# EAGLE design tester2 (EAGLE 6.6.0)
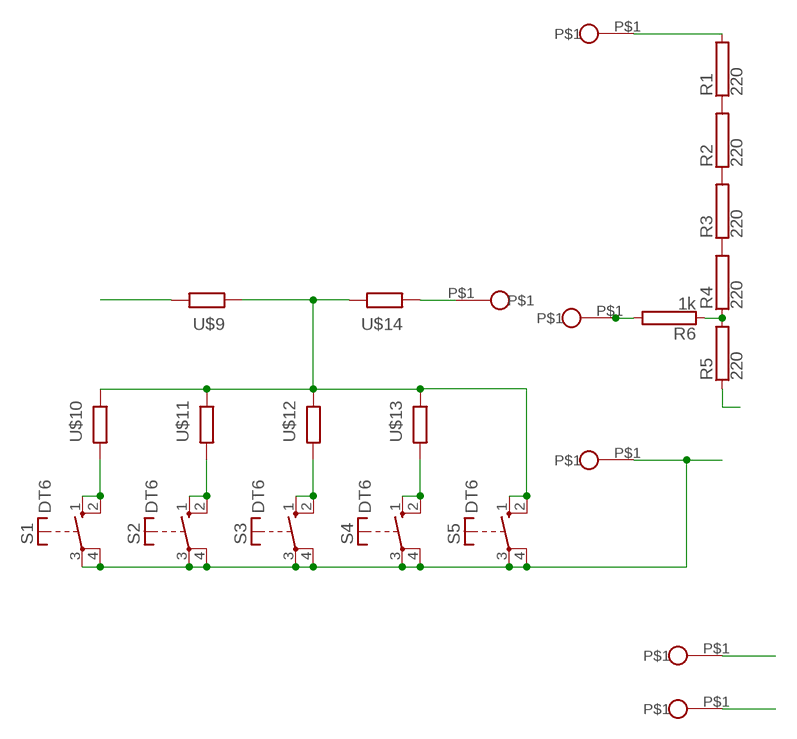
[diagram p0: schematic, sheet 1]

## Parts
R1  220  RCA5220  [CA5220]
R2  220  RCA5220  [CA5220]
R3  220  RCA5220  [CA5220]
R4  220  RCA5220  [CA5220]
R5  220  RCA5220  [CA5220]
R6  1k  RHPS923  [HPS923]
S1  DT6  [DT6]
S2  DT6  [DT6]
S3  DT6  [DT6]
S4  DT6  [DT6]
S5  DT6  [DT6]
U$2  PIN_N  [PIN_N]
U$3  PIN_N  [PIN_N]
U$6  PIN_N  [PIN_N]
U$8  PIN_N  [PIN_N]
U$9  R06W  [R06W2]
U$10  R06W  [R06W2]
U$11  R06W  [R06W2]
U$12  R06W  [R06W2]
U$13  R06W  [R06W2]
U$14  R06W  [R06W2]
U$16  PIN_N  [PIN_N]
U$17  PIN_N  [PIN_N]

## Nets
-UG: U$9.2
F1: U$16.P$1
F2: U$17.P$1
GND: S1.3(P) S1.4(P) S2.3(P) S2.4(P) S3.3(P) S3.4(P) S4.3(P) S4.4(P) S5.3(P) S5.4(P) U$6.P$1
N$1: R1.1 R2.2
N$2: R2.1 R3.2
N$3: R3.1 R4.2
N$4: R4.1 R5.2 R6.1
N$11: S1.1(S) S1.2(S) U$10.1
N$14: S2.1(S) S2.2(S) U$11.1
N$15: S3.1(S) S3.2(S) U$12.1
N$16: S4.1(S) S4.2(S) U$13.1
N$29: S5.1(S) S5.2(S) U$9.1 U$10.2 U$11.2 U$12.2 U$13.2 U$14.2
UA: R1.2 U$3.P$1
UB: R5.1
UG1: U$8.P$1 U$14.1
UG2: R6.2 U$2.P$1

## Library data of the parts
R1-R6 = resistor-power:R: Power Resitor; OC_FARNELL: unknown; OC_NEWARK: unknown
S1-S5 = switch-misc:DT: ITT SWITCH
U$2 U$3 U$6 U$8 U$16 U$17 = lampy02:PIN_N
U$9-U$14 = lampy02:R06W

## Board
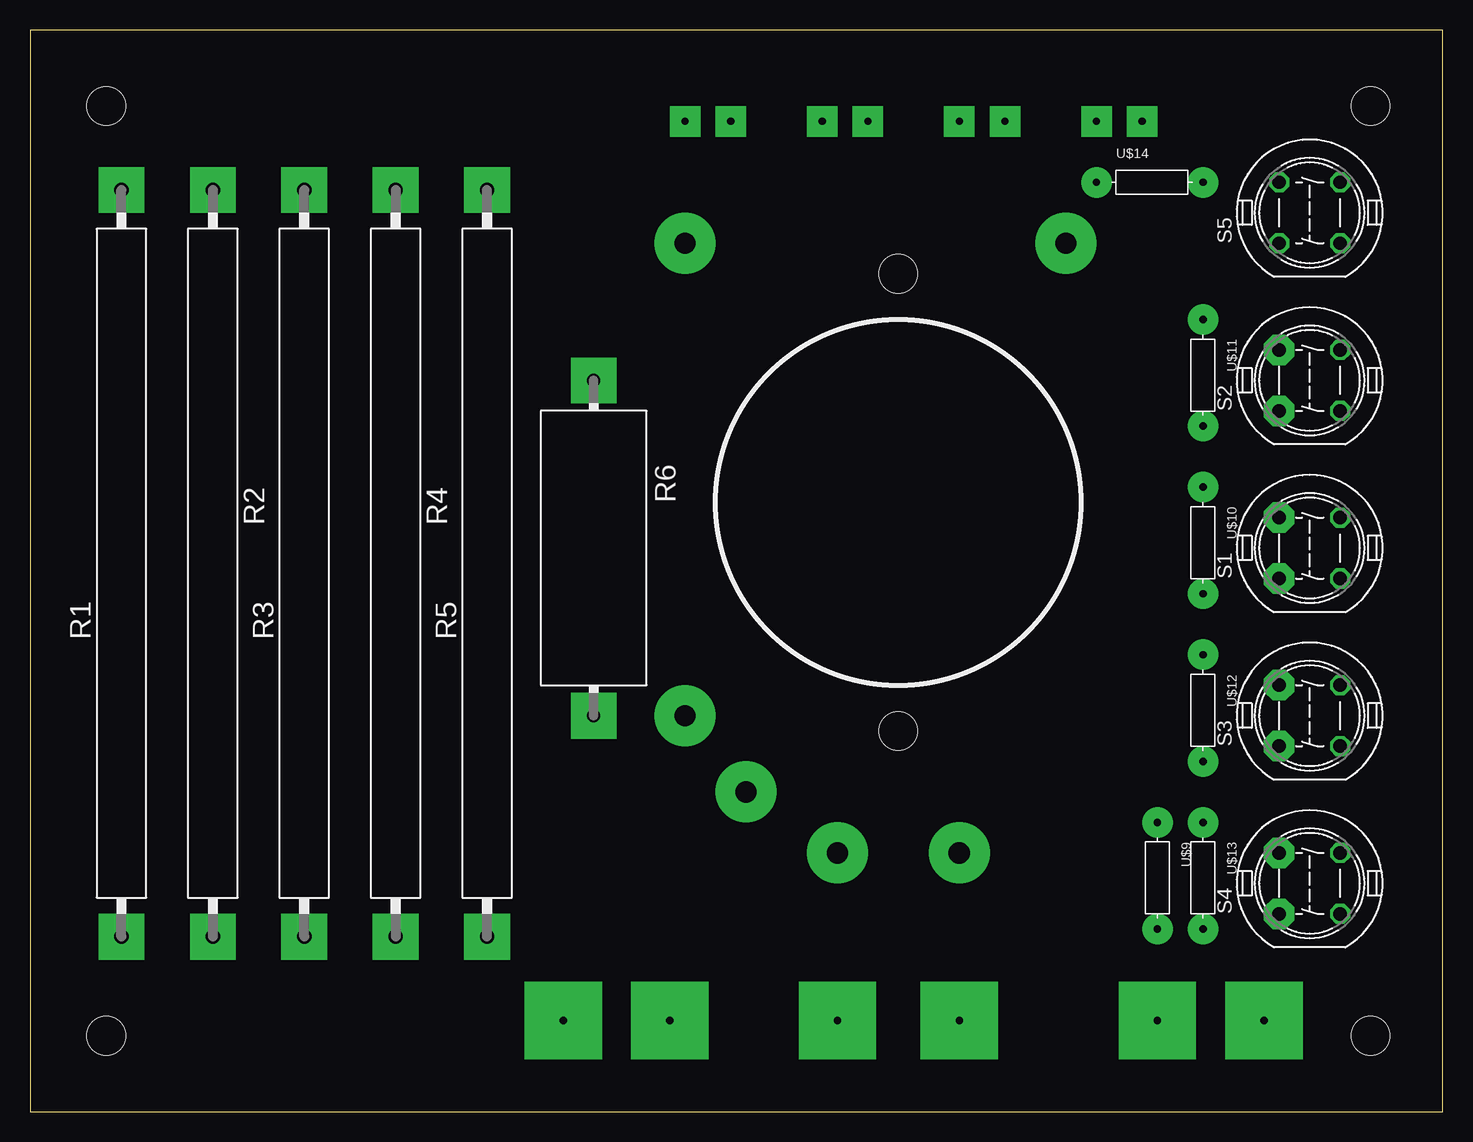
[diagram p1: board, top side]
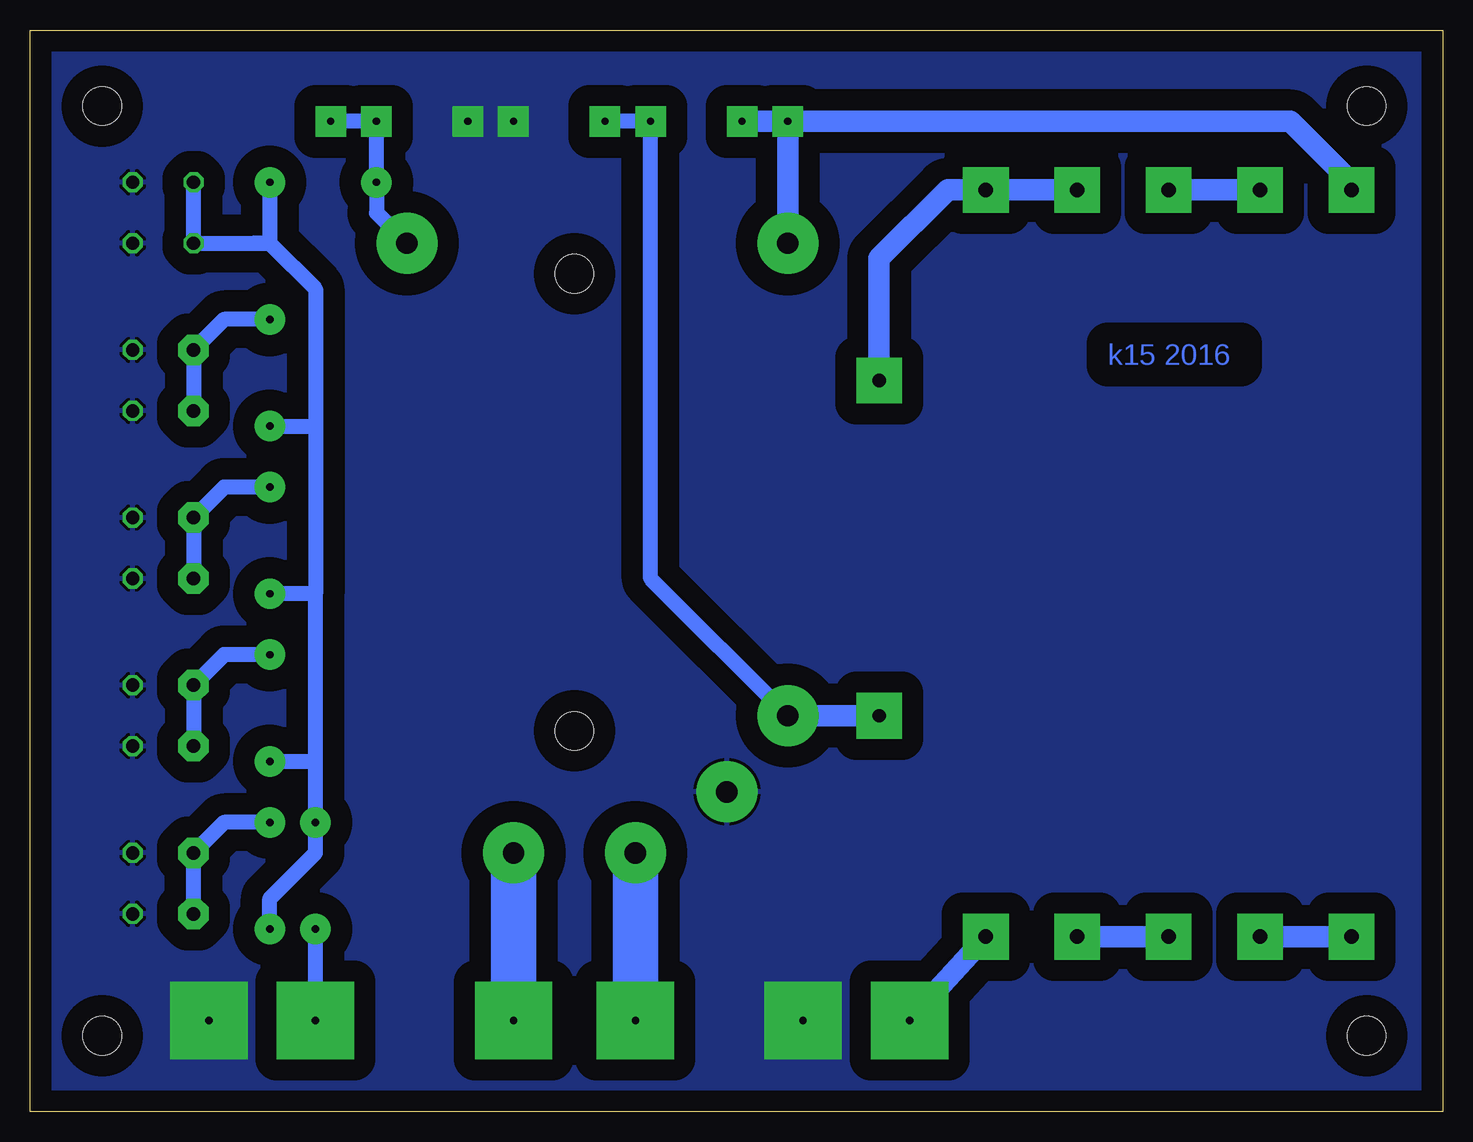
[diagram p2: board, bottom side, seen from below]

Size 117.78 x 90.16 mm. Coordinates in mm from the lower left corner, seen from the top.
Outline: 0,0 117.78,0 117.78,90.16 0,90.16 0,0
Copper layers (1*16): Top 0.035mm / dielectric 1.5mm / Bottom 0.035mm
Design rules "default": minimum track width 10mil, minimum drill 24mil, track to track 8mil, track to pad 8mil, pad to pad 8mil, via to via 8mil, smd to smd 8mil, copper to edge 40mil, drill to drill 8mil, minimum pad ring 10mil, minimum via ring 8mil, stop-mask expansion 4mil, vias tented up to drill 0mil, thermal gap 10mil
Holes 3.2 mm at 72.39,31.75 72.39,69.85 6.35,6.35 6.35,83.82 111.76,83.82 111.76,6.35

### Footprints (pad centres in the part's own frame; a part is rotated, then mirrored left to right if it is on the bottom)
CA5220 = drill 1.2 pad 2: 1 -31.115,0; 2 31.115,0
HPS923 = drill 1.1 pad 1.7: 1 -13.97,0; 2 13.97,0
DT6 = drill 1.118 octagon: 1 -2.54,2.54; 2 2.54,2.54; 3 2.54,-2.54; 4 -2.54,-2.54
PIN_N = drill 1.778 pad 5.08: P$1 0,0
R06W2 = drill 0.61 pad 2.54: 1 -3.81,0; 2 5.079,0

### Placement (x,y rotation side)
R1  7.62,45.72 90 top
R2  15.24,45.72 270 top
R3  22.86,45.72 90 top
R4  30.48,45.72 270 top
R5  38.1,45.72 90 top
R6  46.99,46.99 270 top
S1  106.68,46.99 90 top
S2  106.68,60.96 90 top
S3  106.68,33.02 90 top
S4  106.68,19.05 90 top
S5  106.68,74.93 90 top
U$2  54.61,33.02 0 top
U$3  54.61,72.39 0 top
U$6  59.69,26.67 0 top
U$8  86.36,72.39 0 top
U$9  93.98,20.32 270 top
U$10  97.79,48.26 270 top
U$11  97.79,62.23 270 top
U$12  97.79,34.29 270 top
U$13  97.79,20.32 270 top
U$14  92.71,77.47 0 top
U$16  77.47,21.59 0 top
U$17  67.31,21.59 0 top

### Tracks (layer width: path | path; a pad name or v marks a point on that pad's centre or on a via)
-UG  (via drill 0.6 pad 6.45)
  Bottom 1.27: v93.98,7.62 U$9.2
F1  (via drill 0.6 pad 6.45)
  Bottom 3.81: v77.47,7.62 U$16.P$1
F2  (via drill 0.6 pad 6.45)
  Bottom 3.81: v67.31,7.62 U$17.P$1
GND  (via drill 0.6 pad 2.54, 0.6 pad 6.45)
  other vias: 53.34,7.62 102.87,7.62 77.47,82.55 81.28,82.55
  pour Bottom (isolate 1.778): 0,90.17 118.11,90.17 118.11,0 0,0
N$1
  Bottom 1.778: R2.2 R1.1
N$2
  Bottom 1.778: R3.2 R2.1
N$3
  Bottom 1.778: R4.2 R3.1
N$4
  Bottom 1.778: R4.1 R5.2 41.27,76.84 46.99,71.12 R6.1
N$5  (via drill 0.6 pad 3.81)
  other vias: 46.99,60.96
N$6  (via drill 0.6 pad 3.81)
  other vias: 7.62,76.84
N$7  (via drill 0.6 pad 3.81)
  other vias: 15.24,76.84
N$8  (via drill 0.6 pad 3.81)
  other vias: 22.86,76.84
N$10  (via drill 0.6 pad 3.81)
  other vias: 30.48,76.84
N$11
  Bottom 1.27: U$10.1 101.6,52.07 S1.2 S1.1
N$12  (via drill 0.6 pad 3.81)
  other vias: 38.1,76.84
N$13  (via drill 0.6 pad 3.81)
  other vias: 7.62,14.6
N$14
  Bottom 1.27: U$11.1 101.6,66.04 S2.2 S2.1
N$15
  Bottom 1.27: U$12.1 101.6,38.1 S3.2 S3.1
N$16
  Bottom 1.27: S4.1 S4.2 101.6,24.13 U$13.1
N$17  (via drill 0.6 pad 3.81)
  other vias: 15.24,14.6
N$18  (via drill 0.6 pad 3.81)
  other vias: 22.86,14.6
N$19  (via drill 0.6 pad 3.81)
  other vias: 30.48,14.6
N$20  (via drill 0.6 pad 3.81)
  other vias: 38.1,14.6
N$21  (via drill 0.6 pad 2.54)
  other vias: 104.14,44.45
N$22  (via drill 0.6 pad 2.54)
  other vias: 104.14,49.53
N$23  (via drill 0.6 pad 2.54)
  other vias: 104.14,35.56
N$24  (via drill 0.6 pad 2.54)
  other vias: 104.14,30.48
N$25  (via drill 0.6 pad 2.54)
  other vias: 104.14,63.5
N$26  (via drill 0.6 pad 2.54)
  other vias: 104.14,58.42
N$27  (via drill 0.6 pad 2.54)
  other vias: 104.14,21.59
N$28  (via drill 0.6 pad 2.54)
  other vias: 104.14,16.51
N$29
  Bottom 1.016: 93.98,43.18 | U$10.2 | 93.98,29.21
  Bottom 1.27: U$13.2 | U$13.2 | U$13.2 97.79,17.78 93.98,21.59 U$9.1 93.98,29.21 U$12.2 | 93.98,29.21 93.98,43.18 | U$10.2 93.98,43.18 93.98,57.15 | U$11.2 93.98,57.15 | 99.06,72.39 S5.1 S5.2 | 99.06,72.39 97.79,72.39 93.98,68.58 93.98,57.15 | U$14.2 97.79,72.39 99.06,72.39
UA  (via drill 0.6 pad 2.54)
  Bottom 1.778: U$3.P$1 v54.61,82.55 | v54.61,82.55 v58.42,82.55 | R1.2 7.62,77.47 12.7,82.55 v54.61,82.55
UB  (via drill 0.6 pad 6.45)
  Bottom 1.778: v44.45,7.62 R5.1
UG1  (via drill 0.6 pad 2.54)
  Bottom 1.27: v92.71,82.55 v88.9,82.55 U$14.1 88.9,74.93 U$8.P$1
UG2  (via drill 0.6 pad 2.54, 0.6 pad 3.81)
  Bottom 1.27: v69.85,82.55 v66.04,82.55 66.04,44.45 U$2.P$1
  Bottom 1.778: R6.2 U$2.P$1
  other vias: 46.99,33.02

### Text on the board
Bottom: k15 2016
